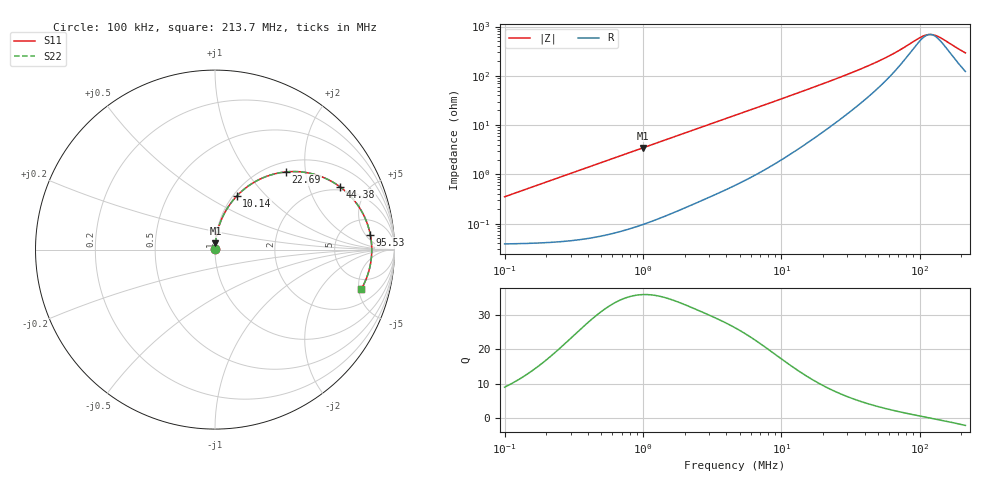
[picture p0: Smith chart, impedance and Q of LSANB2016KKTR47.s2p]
! LSANB2016KKTR47  S-PARAMETER MODEL  ( General Type )
! Model Generated by TAIYO YUDEN Corporation (http://www.ty-top.com)
! Version 3.0
! TAIYO YUDEN Control No. 20210629
! Copyright(c) 2013 TAIYO YUDEN CO.,LTD. All Rights Reserved.
! Product Description (link to TY-COMPAS)
! https://ds.yuden.co.jp/TYCOMPAS/or/detail?pn=LSANB2016KKTR47M&u=M
! Products Name : Inductors
! Characteristics :
!  Inductance : 0.47 uH , SRF(min) : -Hz , DC Resistance(max) : 0.046 Ohm
!  Rated Current : Saturation :3200 mA , Temp Rise : 2800 mA (40 degC)
!  Case Size : 2.0 x 1.6 / 0.079 x 0.063 [mm/inch] , Thickness : 1 / 0.039 [mm/inch]
!  (Conditions: Temperature = 25 degC , DC Bias Current/Voltage = 0A / 0V)
! External Node Assignments :
!  1  o---GGG---o  2
! GND o---------o GND
! Frequency Range : 0.1MHz  -  213.673535MHz  [ 402 STEP ]
# MHz S RI R 50
! Freq[MHz].  S11 Real  S11 Imag  S21 Real  S21 Imag  S12 Real  S12 Imag  S22 Real  S22 Imag
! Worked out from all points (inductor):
!   401 points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, 100 kHz to 213.7 MHz, reference 50 ohm
!   read as one part in series: L = 555 nH near 103.9 kHz
!   highest Q = 36 at 997.5 kHz (marker M1), where L = 551 nH
!   self-resonance near 118.7 MHz
!   S11 on the Smith chart (normalised r, x): 100 kHz: 1.00, +0.01; 10.14 MHz: 1.04, +0.69; 22.69 MHz: 1.19, +1.57; 44.38 MHz: 1.83, +3.27; 95.53 MHz: 10, +7; 213.7 MHz: 3.45, -5.30
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0.1  0.0004 0.00349  0.9996 -0.00349  0.9996 -0.00349  0.0004 0.00349
0.361188  0.000637 0.0126  0.9994 -0.0126  0.9994 -0.0126  0.000637 0.0126
0.997528  0.00215 0.0344  0.9979 -0.0344  0.9979 -0.0344  0.00215 0.0344
1.304567  0.00328 0.0449  0.9967 -0.0449  0.9967 -0.0449  0.00328 0.0449
2.601022  0.0107 0.0879  0.9893 -0.0879  0.9893 -0.0879  0.0107 0.0879
4.71194  0.0307 0.1544  0.9693 -0.1544  0.9693 -0.1544  0.0307 0.1544
7.183499  0.0655 0.2252  0.9345 -0.2252  0.9345 -0.2252  0.0655 0.2252
10.1432  0.1201 0.2971  0.8799 -0.2971  0.8799 -0.2971  0.1201 0.2971
13.01343  0.1816 0.3514  0.8184 -0.3514  0.8184 -0.3514  0.1816 0.3514
16.69585  0.2653 0.3992  0.7347 -0.3992  0.7347 -0.3992  0.2653 0.3992
22.68813  0.3961 0.4329  0.6039 -0.4329  0.6039 -0.4329  0.3961 0.4329
31.42773  0.5504 0.4202  0.4496 -0.4202  0.4496 -0.4202  0.5504 0.4202
44.37638  0.6973 0.3492  0.3027 -0.3492  0.3027 -0.3492  0.6973 0.3492
60.30341  0.7925 0.2521  0.2075 -0.2521  0.2075 -0.2521  0.7925 0.2521
74.45777  0.8358 0.1762  0.1642 -0.1762  0.1642 -0.1762  0.8358 0.1762
95.52717  0.8653 0.0827  0.1347 -0.0827  0.1347 -0.0827  0.8653 0.0827
111.3581  0.8727 0.0244  0.1273 -0.0244  0.1273 -0.0244  0.8727 0.0244
117.9492  0.8734 0.00255  0.1266 -0.00255  0.1266 -0.00255  0.8734 0.00255
127.3481  0.8727 -0.0267  0.1273 0.0267  0.1273 0.0267  0.8727 -0.0267
142.8693  0.868 -0.0704  0.132 0.0704  0.132 0.0704  0.868 -0.0704
190.4603  0.8358 -0.179  0.1642 0.179  0.1642 0.179  0.8358 -0.179
213.6735  0.8142 -0.2213  0.1858 0.2213  0.1858 0.2213  0.8142 -0.2213
